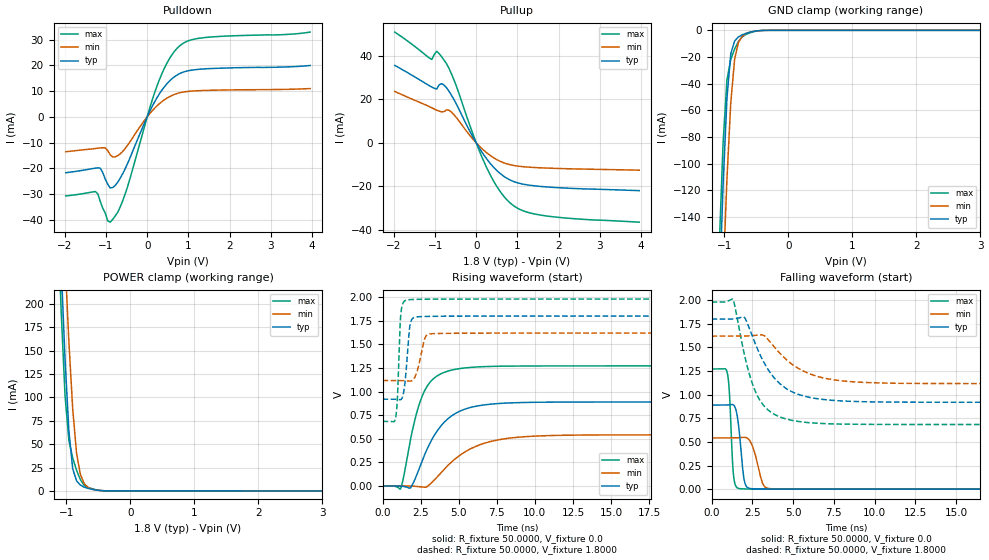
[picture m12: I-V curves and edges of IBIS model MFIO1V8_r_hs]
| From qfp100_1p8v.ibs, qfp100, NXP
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[Model] MFIO1V8_r_hs
|   Model MFIO1V8_r_hs
| This model was characterised for following simulation conditions:
| External (pad) voltage:
|   - Typ: 1.8V,   - Min: 1.62V,   - Max: 1.98V
| Library cells for typ/min/max conditions are connected as defined below:
|  IO - External Pad
|  A - Core Input
|  EN - Output Buffer Enable
|  BOOST - vdde
|  EHS - vdd
|  ENZI - vdd
|  EPD - vdd
|  EPUN - gnd
|  ZI - NC
|  ZIF - NC
|  gnd - gnd
|  gnde - gnde
|  vdd - vdd
|  vdde - vdde
| All other pins connected to ground
Model_type I/O
Polarity   Non-Inverting
Enable   Active-Low
Vinl =   0.5400V
Vinh =   1.2600V
Vmeas =  0.9000V
Cref =   0.0F
Rref =   100.0000
Vref =   0.0V
C_comp   1.5958pF   1.5126pF   1.6704pF
|C_comp_pullup   0.7898pF   0.8219pF   0.7460pF
|C_comp_pulldown   0.5931pF   0.6315pF   0.5575pF
[Model Spec]
| variable   typ   min   max
Vinh   0.5400V   0.4860V   0.5940V
Vinl   1.2600V   1.1340V   1.3860V
Vmeas   0.9000V   0.8100V   0.9900V
[Temperature Range]   25.0000   0.1250k   -40.0000
[Voltage Range]   1.8000V   1.6200V   1.9800V
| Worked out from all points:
|   slope of the pulldown table from 0 to 0.27 V, typ, clamps not added: 32.6 ohm
|   slope of the pullup table from 0 to 0.27 V, typ, clamps not added: 34.8 ohm
|   GND clamp passes 1 mA (typ) near -0.56 V on its own axis
|   POWER clamp passes 1 mA (typ) near -0.54 V on its own axis
|   rising waveform, R_fixture 50.0000, V_fixture 0.0: 20-80 % time 1.9ns typ, 2.67ns min, 1.22ns max; typ from 0 V to 0.89 V
|   rising waveform, R_fixture 50.0000, V_fixture 1.8000: 20-80 % time 265ps typ, 418ps min, 177ps max; typ from 0.92 V to 1.8 V
|   falling waveform, R_fixture 50.0000, V_fixture 0.0: 20-80 % time 304ps typ, 487ps min, 201ps max; typ from 0.89 V to 0 V
|   falling waveform, R_fixture 50.0000, V_fixture 1.8000: 20-80 % time 1.84ns typ, 2.29ns min, 1.29ns max; typ from 1.8 V to 0.92 V
[Pulldown]
|Voltage   I(typ)   I(min)   I(max)
-1.98V    -21.74mA   -13.58mA   -30.76mA
-1.26V    -19.96mA   -12.33mA   -29.04mA
-1.14V    -19.96mA   -12.1mA    -33mA
-960mV    -26.19mA   -13.15mA   -40.44mA
-840mV    -27.51mA   -15.58mA   -39.92mA
-540mV    -20.34mA   -12.41mA   -30.2mA
60mV      2.086mA    1.197mA    3.341mA
300mV     9.043mA    5.145mA    14.58mA
540mV     13.88mA    7.813mA    22.59mA
840mV     17.16mA    9.517mA    28.23mA
1.44V     18.67mA    10.27mA    30.87mA
3.96V     19.95mA    10.98mA    32.93mA
[Pullup]
|Voltage   I(typ)   I(min)   I(max)
-1.98V    35.7mA     23.68mA    51.03mA
-1.08V    25.71mA    16.17mA    38.42mA
-960mV    24.81mA    15.04mA    42.18mA
-840mV    27.29mA    14.27mA    39.65mA
-720mV    25.36mA    15.21mA    36.42mA
-540mV    19.88mA    12.94mA    28.95mA
-60mV     2.001mA    1.263mA    3.041mA
240mV     -7.02mA    -4.333mA   -10.88mA
600mV     -14.41mA   -8.644mA   -22.88mA
900mV     -17.74mA   -10.36mA   -28.83mA
1.74V     -20.33mA   -11.62mA   -33.75mA
3.96V     -22mA      -12.58mA   -36.53mA
[GND_clamp]
|Voltage   I(typ)   I(min)   I(max)
-1.98V    -1.781A    -1.801A    -1.77A
-1.08V    -200.1mA   -270.2mA   -162.2mA
-1.02V    -116mA     -186.2mA   -84.49mA
-960mV    -51.26mA   -111.8mA   -37.36mA
-900mV    -17.65mA   -54.44mA   -21.7mA
-840mV    -8.02mA    -21.7mA    -14.08mA
-780mV    -4.924mA   -8.964mA   -8.313mA
-720mV    -3.338mA   -4.442mA   -4.753mA
-600mV    -1.403mA   -1.338mA   -1.896mA
-480mV    -330.4uA   -347.3uA   -423.3uA
-360mV    -26.82uA   -39.45uA   -30.02uA
3.96V     0A         0A         0A
[POWER_clamp]
|Voltage   I(typ)   I(min)   I(max)
-1.98V    2.119A     2.147A     2.105A
-1.14V    349.2mA    450mA      300.6mA
-1.08V    239.1mA    345.9mA    191.2mA
-1.02V    140.4mA    247.8mA    101.7mA
-960mV    64.08mA    159.3mA    53.89mA
-900mV    23.59mA    87.23mA    35.11mA
-840mV    10.79mA    40.2mA     22.07mA
-780mV    6.218mA    17.5mA     11.92mA
-720mV    4.013mA    7.752mA    6.009mA
-600mV    1.739mA    1.846mA    2.368mA
-360mV    67.5uA     96.07uA    73.34uA
3.96V     0A         0A         0A
[Ramp]
| variable   typ   min   max
dV/dt_r  0.5338/1.8980n   0.3252/2.6729n   0.7629/1.2216n
dV/dt_f  0.5279/1.8402n   0.3013/2.2896n   0.7771/1.2859n
R_load = 50.0000
[Rising Waveform]
R_fixture= 50.0000
V_fixture= 0.0
V_fixture_min= 0.0
V_fixture_max= 0.0
|time   V(typ)   V(min)   V(max)
0s        1.134nV    103.8nV    53.92pV
1.185ns   -400uV     61.59uV    -28.39mV
1.81ns    -22.12mV   -52.04uV   470.8mV
2.197ns   98.35mV    -3.459mV   749.4mV
3.085ns   445mV      15.01mV    1.093V
4.245ns   706.4mV    209.9mV    1.214V
5.833ns   834.5mV    398.3mV    1.257V
8.342ns   879.9mV    507.3mV    1.27V
12.89ns   889.4mV    539.5mV    1.272V
100ns     889.7mV    541.9mV    1.272V
[Rising Waveform]
R_fixture= 50.0000
V_fixture= 1.8000
V_fixture_min= 1.6200
V_fixture_max= 1.9800
|time   V(typ)   V(min)   V(max)
0s        919.5mV    1.117V     684.3mV
849.4ps   919.7mV    1.117V     715.3mV
965ps     917.4mV    1.117V     898.2mV
1.132ns   912.8mV    1.118V     1.637V
1.225ns   917.9mV    1.118V     1.856V
1.461ns   1.076V     1.115V     1.961V
1.787ns   1.688V     1.11V      1.973V
2.827ns   1.796V     1.582V     1.978V
3.448ns   1.797V     1.614V     1.978V
100ns     1.799V     1.619V     1.979V
[Falling Waveform]
R_fixture= 50.0000
V_fixture= 0.0
V_fixture_min= 0.0
V_fixture_max= 0.0
|time   V(typ)   V(min)   V(max)
0s        889.7mV    541.9mV    1.272V
964.1ps   890.1mV    542mV      1.231V
1.092ns   892.4mV    541.9mV    1.028V
1.358ns   889.2mV    541.7mV    130mV
1.587ns   764mV      543mV      12.78mV
1.811ns   402.6mV    546.4mV    4.056mV
2.162ns   24.44mV    542.6mV    1.967mV
3.181ns   1.567mV    44.58mV    612.1uV
3.791ns   888.3uV    3.3mV      343.7uV
100ns     11.12nV    119.5nV    6.009nV
[Falling Waveform]
R_fixture= 50.0000
V_fixture= 1.8000
V_fixture_min= 1.6200
V_fixture_max= 1.9800
|time   V(typ)   V(min)   V(max)
0s        1.799V     1.619V     1.979V
1.329ns   1.8V       1.619V     2.002V
1.992ns   1.819V     1.619V     1.442V
2.315ns   1.703V     1.622V     1.219V
2.73ns    1.519V     1.628V     1.017V
3.209ns   1.342V     1.626V     882.4mV
4.431ns   1.083V     1.396V     750mV
6.344ns   960.8mV    1.201V     698.6mV
13.28ns   919.8mV    1.118V     684.2mV
100ns     919.5mV    1.117V     684.3mV
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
